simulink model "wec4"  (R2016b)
settings: Solver=ode4  StartTime=0  StopTime=1000  FixedStep=0.005  MaxStep=0.005  RelTol=1e-3  EnableMultiTasking=on
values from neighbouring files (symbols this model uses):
  arAdaptiveLawData = 1/2*zModelSimple.zModelPto.arFreq.*     zModelSimple.zModelPto.arMagnitude./     cos(zModelSimple.zModelPto.arPhase*pi/180+pi/2)    [IMPACT_Control.m]
  arAdaptiveLawDataX = 1/2*zModelSimpleX.zModelPto.arFreq.*         zModelSimpleX.zModelPto.arMagnitude./         cos(zModelSimpleX.zModelPto.arPhase*pi/180+pi/2)    [IMPACT_Control.m]
  arControllerRampGain = [0,0,1,1]    [IMPACT_Control.m]
  arControllerRampTime = [0 rStartRampTime rStartRampTime+rRampTimeLength 8000]    [IMPACT_Control.m]
  arEkfInitialisation = zeros(1,11)    [IMPACT_Control.m]
  arEkfInitialisationX = zeros(1,11)    [IMPACT_Control.m]
  arFrequency = zModelSimple.zModelPto.arFreq    [IMPACT_Control.m]
  arFrequencyRange = zModelSimple.zModelPto.arFreq    [IMPACT_Control.m]
  arFrequencyX = zModelSimpleX.zModelPto.arFreq    [IMPACT_Control.m]
  arImpedance = 1./zModelSimple.zModelPto.arMagnitude./zModelSimple.zModelPto.arFreq    [IMPACT_Control.m]
  arImpedanceX = 1./zModelSimpleX.zModelPto.arMagnitude./zModelSimpleX.zModelPto.arFreq    [IMPACT_Control.m]
  CentralPTOPreload = -1.6113e+07    (= -16113000)    [wecSimInputFile.m]
  F1 = [4.243 2.375 -12.243]    [wecSimInputFile.m]
  F2 = [4.243 -2.375 -12.243]    [wecSimInputFile.m]
  F3 = [-4.243 -2.375 -12.243]    [wecSimInputFile.m]
  F4 = [-4.243 2.375 -12.243]    [wecSimInputFile.m]
  FC = [0 0 -14]    [wecSimInputFile.m]
  iAdaptiveDamping = 0    [wec4IMPACT_Project.m]    (also in IMPACT_Control.m = handles.iAdaptiveDamping; wec1_IMPACT_Project.m; wec2_IMPACT_Project.m; wec3_IMPACT_Project.m)
  iControlType = 2    [wec4IMPACT_Project.m]    (also in IMPACT_Control.m = handles.iControlType; wec1_IMPACT_Project.m = 1; wec2_IMPACT_Project.m = 1; wec3_IMPACT_Project.m = 1)
  iPtoPositionConstraint = 1    [wec4IMPACT_Project.m]    (also in IMPACT_Control.m = handles.iPtoPositionConstraint; wec1_IMPACT_Project.m = 0; wec2_IMPACT_Project.m; wec3_IMPACT_Project.m)
  iSensorNoise = 0    [IMPACT_Control.m]
  m = m+1    (= 2)    [checkParamFile.m]
  PTOrotation = atan((T1(2)-F1(2))/(T1(1)-F1(1)))    [wecSimInputFile.m]
  rCogFloater = -8    [wec4_IMPACT_Model.m]    (also in paramInitial.m = get( handles.edit_rCogFloater, 'String' ); wec1_IMPACT_Model.m = -18; wec2_IMPACT_Model.m = -8.5; wec3_IMPACT_Model.m = -0.7)
  rCogSpar = -36.6    [wec4_IMPACT_Model.m]    (also in paramInitial.m = get( handles.edit_rCogSpar, 'String' ); wec3_IMPACT_Model.m = -21.3; wec3_IMPACT_Model2.m = -21.3)
  rDisplacementLimit = 10.000000    (= 10)    [wec4IMPACT_Project.m]    (also in IMPACT_Control.m = getValue(handles.edit_displacementLimit); wec1_IMPACT_Project.m; wec2_IMPACT_Project.m; wec3_IMPACT_Project.m = 3)
  rDisplacementLimitX = 10.000000    (= 10)    [wec4IMPACT_Project.m]    (also in IMPACT_Control.m = getValue(handles.edit_displacementLimitX); wec1_IMPACT_Project.m = 0; wec2_IMPACT_Project.m; wec3_IMPACT_Project.m = 0)
  rGainForAntiWIndUp = tfControllerDiscrete.rGain    [IMPACT_Control.m]
  rGainForAntiWIndUpX = tfControllerXDiscrete.rGain    [IMPACT_Control.m]
  rMaxForcePto = 300000000.000000    (= 300000000)    [wec4IMPACT_Project.m]    (also in IMPACT_Control.m = getValue(handles.edit_maxForcePto); wec1_IMPACT_Project.m = 1e+15; wec2_IMPACT_Project.m = 1e+15; wec3_IMPACT_Project.m = 1000000000)
  rMinForcePto = -300000000.000000    (= -300000000)    [wec4IMPACT_Project.m]    (also in IMPACT_Control.m = getValue(handles.edit_minForcePto); wec1_IMPACT_Project.m = -1e+15; wec2_IMPACT_Project.m = -1e+15; wec3_IMPACT_Project.m = -1000000000)
  rMooringX = 20000    [wec4_IMPACT_Model.m]    (also in paramInitial.m = get( handles.edit_rMooringX, 'String' ); wec3_IMPACT_Model.m = 10000; wec3_IMPACT_Model2.m = 10000)
  rMooringZ = 10000    [wec4_IMPACT_Model.m]    (also in paramInitial.m = get( handles.edit_rMooringZ, 'String' ); wec3_IMPACT_Model.m = 0; wec3_IMPACT_Model2.m = 0)
  rOutputSampleTime = 0.010000    (= 0.01)    [wec4IMPACT_Project.m]    (also in IMPACT_Control.m = getValue(handles.edit_outputSampleTime); wec1_IMPACT_Project.m; wec2_IMPACT_Project.m; wec3_IMPACT_Project.m)
  rPassiveDampingGain = -604830.000000    (= -604830)    [wec4IMPACT_Project.m]    (also in IMPACT_Control.m = getValue(handles.edit_gainPLD); wec1_IMPACT_Project.m = -214018.1537; wec2_IMPACT_Project.m = -1948070; wec3_IMPACT_Project.m = -519390)
  rPassiveDampingGainX = -278660.000000    (= -278660)    [wec4IMPACT_Project.m]    (also in IMPACT_Control.m = getValue(handles.edit_gainPLDX); wec1_IMPACT_Project.m = 0; wec2_IMPACT_Project.m = 0; wec3_IMPACT_Project.m = 0)
  rTetherPretension = 1.6113e+07    (= 16113000)    [wec4_IMPACT_Model.m]    (also in paramInitial.m = get( handles.edit_rTetherPretension, 'String' ); wec3_IMPACT_Model.m = 0; wec3_IMPACT_Model2.m = 0)
  rTetherSpring = 500000    [wec4_IMPACT_Model.m]    (also in paramInitial.m = get( handles.edit_rTetherSpring, 'String' ); wec3_IMPACT_Model.m = 0; wec3_IMPACT_Model2.m = 0)
  rUpperFrequencyLimit = EKFFloater.upperFreq    [IMPACT_Control.m]
  rXf = 4.243    [wec4AdditionalParams.m]
  rXs = 16.075    [wec4AdditionalParams.m]
  rYf = 2.375    [wec4AdditionalParams.m]
  rYs = 16.075    [wec4AdditionalParams.m]
  rZf = 4.243    [wec4AdditionalParams.m]
  rZs = 2.4350    (= 2.435)    [wec4AdditionalParams.m]
  rZTetherF = 6    [wec4AdditionalParams.m]
  rZTetherS = 2.4350    (= 2.435)    [wec4AdditionalParams.m]
  s = tf('s')    [wec4_IMPACT_Model.m]    (also in IMPACT_Control.m; wec1_IMPACT_Model.m; wec2_IMPACT_Model.m; wec3_IMPACT_Model.m)
  SidePTO1Preload = PreloadPTOCorner    (= 0)    [wecSimInputFile.m]
  SidePTO2Preload = PreloadPTOCorner    (= 0)    [wecSimInputFile.m]
  SidePTO3Preload = PreloadPTOCorner    (= 0)    [wecSimInputFile.m]
  SidePTO4Preload = PreloadPTOCorner    (= 0)    [wecSimInputFile.m]
  simu = simulationClass()    [wecSimInputFile.m]
  T1 = [16.075 16.075 -34.165]    [wecSimInputFile.m]
  T2 = [16.075 -16.075 -34.165]    [wecSimInputFile.m]
  T3 = [-16.075 -16.075 -34.165]    [wecSimInputFile.m]
  T4 = [-16.075 16.075 -34.165]    [wecSimInputFile.m]
  TC = [0 0 -34.165]    [wecSimInputFile.m]
  waves = waveClass('irregular')    [wecSimInputFile.m]
  Z = magPhaseToComplex(zModelTf)    [IMPACT_Control.m]
undefined symbols (not defined in the file or in its folder): arControllerDiscreteDen, arControllerDiscreteNum, arControllerDiscreteXDen, arControllerDiscreteXNum, arExcForceFloaterDen, arExcForceFloaterNum, arExcForceFloaterXDen, arExcForceFloaterXNum, arExcForceSparDen, arExcForceSparNum, arExcForceSparXDen, arExcForceSparXNum, arFexcFloaterDen, arFexcFloaterNum, arFexcFloaterXDen, arFexcFloaterXNum, arFexcSparDen, arFexcSparNum, arFexcSparXDen, arFexcSparXNum, Body, body, constraint, CTTime, deg, Elements, geometry, IRKB, kg, lenJ, mooring, N, pto, rAccelerationGainFloater, rAccelerationGainFloaterX, rAccelerationGainSpar, rAccelerationGainSparX, rad, rBuoyancyGainFloater, rBuoyancyGainFloaterX, rBuoyancyGainSpar, rBuoyancyGainSparX, rDampingGainFloater, rDampingGainFloaterX, rDampingGainSpar, rDampingGainSparX, Rigid, rMaxFocePto, wec4_float, wec4_reactor, WECSim_Lib, X, Y
libraries: nesl_utility x380, sm_lib x170, vrlib x91, simulink x12, WECSim_Lib x4
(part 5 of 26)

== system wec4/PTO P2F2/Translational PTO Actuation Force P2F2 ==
  Force : Inport
  Assignment{,1..3} (4 alike) : Assignment  IndexOptions=Index vector (dialog)  Indices=3  OutputSizes=1
  Bus Creator2 : BusCreator  Inputs=3
  Constant{,1..3} (4 alike) : Constant  Value=[0 0 0 0 0 0]
  InternalMechanics : Subsystem
  Mux : Mux  Inputs=2
  Mux1 : Mux  Inputs=2
  Mux2 : Mux  Inputs=8
  PS-Simulink Converter{,1..7} (8 alike) : nesl_utility/PS-Simulink Converter  PhysicalDomain=network_engine_domain  SubClassName=ps_output  LeftPortType=input  RightPortType=output  PseudoPeriodic=off  Frequencies=[]  Unit=1  AffineConversion=off
  Rigid Transform (Position) : sm_lib/Frames and Transforms/Rigid Transform  TranslationMethod=Cartesian  TranslationStandardOffset=0  TranslationLengthUnit=m  TranslationStandardAxis=+Z  TranslationCartesianOffset=pto.initDisp.initLinDisp + pto.loc  TranslationROffset=0  TranslationROffsetUnits=m  TranslationZOffset=0  TranslationZOffsetUnits=m  TranslationThetaOffset=0  TranslationThetaOffsetUnits=deg  RotationMethod=None  RotationAngleUnits=rad  RotationStandardAxis=+Y  RotationAngle=0  RotationArbitraryAxis=[0 1 0]  FollAlignAxisA=+X  BaseAlignAxisA=+Y  FollAlignAxisB=+Y  BaseAlignAxisB=+Z  RotationSequenceAxes=FollowerAxes  RotationSequence=XYX  RotationSequenceAngles=[0 0 0]  RotationSequenceAnglesUnits=deg  RotationMatrix=[1 0 0; 0 1 0; 0 0 1]
  Rigid Transform (Position)1 : sm_lib/Frames and Transforms/Rigid Transform  TranslationMethod=Cartesian  TranslationStandardOffset=0  TranslationLengthUnit=m  TranslationStandardAxis=+Z  TranslationCartesianOffset=pto.initDisp.initLinDisp + pto.loc  TranslationROffset=0  TranslationROffsetUnits=m  TranslationZOffset=0  TranslationZOffsetUnits=m  TranslationThetaOffset=0  TranslationThetaOffsetUnits=deg  RotationMethod=None  RotationAngleUnits=rad  RotationStandardAxis=+Y  RotationAngle=0  RotationArbitraryAxis=[0 1 0]  FollAlignAxisA=+X  BaseAlignAxisA=+Y  FollAlignAxisB=+Y  BaseAlignAxisB=+Z  RotationSequenceAxes=FollowerAxes  RotationSequence=XYX  RotationSequenceAngles=[0 0 0]  RotationSequenceAnglesUnits=deg  RotationMatrix=[1 0 0; 0 1 0; 0 0 1]
  Rigid Transform (Orientation) : sm_lib/Frames and Transforms/Rigid Transform  TranslationMethod=None  TranslationStandardOffset=0  TranslationLengthUnit=m  TranslationStandardAxis=+Z  TranslationCartesianOffset=0  TranslationROffset=0  TranslationROffsetUnits=m  TranslationZOffset=0  TranslationZOffsetUnits=m  TranslationThetaOffset=0  TranslationThetaOffsetUnits=deg  RotationMethod=RotationMatrix  RotationAngleUnits=rad  RotationStandardAxis=+Y  RotationAngle=0  RotationArbitraryAxis=[0 1 0]  FollAlignAxisA=+X  BaseAlignAxisA=+Y  FollAlignAxisB=+Y  BaseAlignAxisB=+Z  RotationSequenceAxes=FollowerAxes  RotationSequence=XYX  RotationSequenceAngles=[0 0 0]  RotationSequenceAnglesUnits=deg  RotationMatrix=pto.orientation.rotationMatrix
  Rigid Transform (Orientation)1 : sm_lib/Frames and Transforms/Rigid Transform  TranslationMethod=None  TranslationStandardOffset=0  TranslationLengthUnit=m  TranslationStandardAxis=+Z  TranslationCartesianOffset=0  TranslationROffset=0  TranslationROffsetUnits=m  TranslationZOffset=0  TranslationZOffsetUnits=m  TranslationThetaOffset=0  TranslationThetaOffsetUnits=deg  RotationMethod=RotationMatrix  RotationAngleUnits=rad  RotationStandardAxis=+Y  RotationAngle=0  RotationArbitraryAxis=[0 1 0]  FollAlignAxisA=+X  BaseAlignAxisA=+Y  FollAlignAxisB=+Y  BaseAlignAxisB=+Z  RotationSequenceAxes=FollowerAxes  RotationSequence=XYX  RotationSequenceAngles=[0 0 0]  RotationSequenceAnglesUnits=deg  RotationMatrix=pto.orientation.rotationMatrix
  Simulink-PS Converter : nesl_utility/Simulink-PS Converter  PhysicalDomain=network_engine_domain  SubClassName=ps_input  LeftPortType=input  RightPortType=output  PseudoPeriodic=off  Frequencies=[]  NoiseDistribution=none  NoiseParameters=[]  Unit=1  AffineConversion=off  InputFiltering=off  SimscapeFilterOrder=1  InputFilterTimeConstant=0.001  UdotUserProvided=1
  Translational PCC (Prismatic Joint) : sm_lib/Joints/Prismatic Joint  SenseConstraintForce=on  SenseConstraintForceX=off  SenseConstraintForceY=off  SenseConstraintForceZ=off  SenseConstraintTorque=on  SenseConstraintTorqueX=off  SenseConstraintTorqueY=off  SenseConstraintTorqueZ=off  SenseTotalForce=on  SenseTotalForceX=off  SenseTotalForceY=off  SenseTotalForceZ=off  SenseTotalTorque=on  SenseTotalTorqueX=off  SenseTotalTorqueY=off  SenseTotalTorqueZ=off  CompositeWrenchDir=BaseOnFollower  CompositeWrenchFrame=BaseFrame  EquilibriumPosition=0  EquilibriumPositionUnits=m  SpringStiffness=pto.k  SpringStiffnessUnits=N/m  DampingCoefficient=pto.c  DampingCoefficientUnits=N/(m/s)  TorqueActuationMode=InputTorque  MotionActuationMode=ComputedMotion  SensePosition=on  SenseVelocity=on  SenseAcceleration=on  SenseTorqueForce=on  PositionTargetSpecify=off  PositionTargetPriority=High  PositionTargetValue=0  PositionTargetValueUnits=m  VelocityTargetSpecify=off  VelocityTargetPriority=High  VelocityTargetValue=0  VelocityTargetValueUnits=m/s
  output : ToWorkspace  VariableName=pto2_out  SaveFormat=Structure With Time  SampleTime=-1
  F : PMIOPort  Port=1  Side=Right
  B : PMIOPort  Port=2  Side=Left
  Response : Outport
  ptoForce : Outport  Port=2
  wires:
  Bus Creator2/1 -> Response/1
  Assignment/1 -> Mux2/1, Bus Creator2/1, InternalMechanics/1(Position)  "position"
  Assignment1/1 -> Mux2/2, Bus Creator2/2, InternalMechanics/2(Velocity)  "velocity"
  Assignment2/1 -> Mux2/3, Bus Creator2/3  "acceleration"
  Force/1 -> Simulink-PS Converter/1
  Mux2/1 -> output/1
  Mux/1 -> Mux2/6  "forceConstraint"
  Mux1/1 -> Mux2/4  "forceTotal"
  PS-Simulink Converter4/1 -> Mux/1
  PS-Simulink Converter5/1 -> Mux/2
  PS-Simulink Converter6/1 -> Mux1/1
  PS-Simulink Converter7/1 -> Mux1/2
  Constant/1 -> Assignment/1
  PS-Simulink Converter/1 -> Assignment/2
  Constant1/1 -> Assignment1/1
  PS-Simulink Converter1/1 -> Assignment1/2
  Constant2/1 -> Assignment2/1
  PS-Simulink Converter2/1 -> Assignment2/2
  InternalMechanics/1(Force) -> Mux2/7  "forceInternalMechanics"
  InternalMechanics/2(Power) -> Mux2/8  "powerInternalMechanics"
  Constant3/1 -> Assignment3/1
  PS-Simulink Converter3/1 -> Assignment3/2  "forceActuation"
  Assignment3/1 -> ptoForce/1, Mux2/5  "forceActuation"
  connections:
  Rigid Transform (Position)/RConn1 -- Rigid Transform (Orientation)/LConn1
  Rigid Transform (Position)1/RConn1 -- Rigid Transform (Orientation)1/LConn1
  Simulink-PS Converter/RConn1 -- Translational PCC (Prismatic Joint)/LConn2
  Rigid Transform (Orientation)/RConn1 -- Translational PCC (Prismatic Joint)/LConn1
  Rigid Transform (Position)/LConn1 -- B/RConn1
  Translational PCC (Prismatic Joint)/RConn5 -- PS-Simulink Converter3/LConn1
  Translational PCC (Prismatic Joint)/RConn9 -- PS-Simulink Converter7/LConn1
  Rigid Transform (Orientation)1/RConn1 -- Translational PCC (Prismatic Joint)/RConn1
  Translational PCC (Prismatic Joint)/RConn4 -- PS-Simulink Converter2/LConn1
  Translational PCC (Prismatic Joint)/RConn7 -- PS-Simulink Converter5/LConn1
  Translational PCC (Prismatic Joint)/RConn3 -- PS-Simulink Converter1/LConn1
  Rigid Transform (Position)1/LConn1 -- F/RConn1
  Translational PCC (Prismatic Joint)/RConn8 -- PS-Simulink Converter6/LConn1
  Translational PCC (Prismatic Joint)/RConn2 -- PS-Simulink Converter/LConn1
  Translational PCC (Prismatic Joint)/RConn6 -- PS-Simulink Converter4/LConn1

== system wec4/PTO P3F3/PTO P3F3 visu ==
  note: 1) Add Subsystem or Model blocks as valid variant choices. 2) You cannot connect blocks at this level. At simulation, connectivity is automatically determined, based on the active variant and port name matching.
  Hydrodynamic Body : Subsystem  VariantControl=sv_b6_hydroBody
  Non-Hydro Body : Subsystem  VariantControl=sv_b6_nonHydroBody
  Conn : PMIOPort  Port=1  Side=Right

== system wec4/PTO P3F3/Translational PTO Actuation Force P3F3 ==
  Force : Inport
  Assignment{,1..3} (4 alike) : Assignment  IndexOptions=Index vector (dialog)  Indices=3  OutputSizes=1
  Bus Creator2 : BusCreator  Inputs=3
  Constant{,1..3} (4 alike) : Constant  Value=[0 0 0 0 0 0]
  InternalMechanics : Subsystem
  Mux : Mux  Inputs=2
  Mux1 : Mux  Inputs=2
  Mux2 : Mux  Inputs=8
  PS-Simulink Converter{,1..7} (8 alike) : nesl_utility/PS-Simulink Converter  PhysicalDomain=network_engine_domain  SubClassName=ps_output  LeftPortType=input  RightPortType=output  PseudoPeriodic=off  Frequencies=[]  Unit=1  AffineConversion=off
  Rigid Transform (Position) : sm_lib/Frames and Transforms/Rigid Transform  TranslationMethod=Cartesian  TranslationStandardOffset=0  TranslationLengthUnit=m  TranslationStandardAxis=+Z  TranslationCartesianOffset=pto.initDisp.initLinDisp + pto.loc  TranslationROffset=0  TranslationROffsetUnits=m  TranslationZOffset=0  TranslationZOffsetUnits=m  TranslationThetaOffset=0  TranslationThetaOffsetUnits=deg  RotationMethod=None  RotationAngleUnits=rad  RotationStandardAxis=+Y  RotationAngle=0  RotationArbitraryAxis=[0 1 0]  FollAlignAxisA=+X  BaseAlignAxisA=+Y  FollAlignAxisB=+Y  BaseAlignAxisB=+Z  RotationSequenceAxes=FollowerAxes  RotationSequence=XYX  RotationSequenceAngles=[0 0 0]  RotationSequenceAnglesUnits=deg  RotationMatrix=[1 0 0; 0 1 0; 0 0 1]
  Rigid Transform (Position)1 : sm_lib/Frames and Transforms/Rigid Transform  TranslationMethod=Cartesian  TranslationStandardOffset=0  TranslationLengthUnit=m  TranslationStandardAxis=+Z  TranslationCartesianOffset=pto.initDisp.initLinDisp + pto.loc  TranslationROffset=0  TranslationROffsetUnits=m  TranslationZOffset=0  TranslationZOffsetUnits=m  TranslationThetaOffset=0  TranslationThetaOffsetUnits=deg  RotationMethod=None  RotationAngleUnits=rad  RotationStandardAxis=+Y  RotationAngle=0  RotationArbitraryAxis=[0 1 0]  FollAlignAxisA=+X  BaseAlignAxisA=+Y  FollAlignAxisB=+Y  BaseAlignAxisB=+Z  RotationSequenceAxes=FollowerAxes  RotationSequence=XYX  RotationSequenceAngles=[0 0 0]  RotationSequenceAnglesUnits=deg  RotationMatrix=[1 0 0; 0 1 0; 0 0 1]
  Rigid Transform (Orientation) : sm_lib/Frames and Transforms/Rigid Transform  TranslationMethod=None  TranslationStandardOffset=0  TranslationLengthUnit=m  TranslationStandardAxis=+Z  TranslationCartesianOffset=0  TranslationROffset=0  TranslationROffsetUnits=m  TranslationZOffset=0  TranslationZOffsetUnits=m  TranslationThetaOffset=0  TranslationThetaOffsetUnits=deg  RotationMethod=RotationMatrix  RotationAngleUnits=rad  RotationStandardAxis=+Y  RotationAngle=0  RotationArbitraryAxis=[0 1 0]  FollAlignAxisA=+X  BaseAlignAxisA=+Y  FollAlignAxisB=+Y  BaseAlignAxisB=+Z  RotationSequenceAxes=FollowerAxes  RotationSequence=XYX  RotationSequenceAngles=[0 0 0]  RotationSequenceAnglesUnits=deg  RotationMatrix=pto.orientation.rotationMatrix
  Rigid Transform (Orientation)1 : sm_lib/Frames and Transforms/Rigid Transform  TranslationMethod=None  TranslationStandardOffset=0  TranslationLengthUnit=m  TranslationStandardAxis=+Z  TranslationCartesianOffset=0  TranslationROffset=0  TranslationROffsetUnits=m  TranslationZOffset=0  TranslationZOffsetUnits=m  TranslationThetaOffset=0  TranslationThetaOffsetUnits=deg  RotationMethod=RotationMatrix  RotationAngleUnits=rad  RotationStandardAxis=+Y  RotationAngle=0  RotationArbitraryAxis=[0 1 0]  FollAlignAxisA=+X  BaseAlignAxisA=+Y  FollAlignAxisB=+Y  BaseAlignAxisB=+Z  RotationSequenceAxes=FollowerAxes  RotationSequence=XYX  RotationSequenceAngles=[0 0 0]  RotationSequenceAnglesUnits=deg  RotationMatrix=pto.orientation.rotationMatrix
  Simulink-PS Converter : nesl_utility/Simulink-PS Converter  PhysicalDomain=network_engine_domain  SubClassName=ps_input  LeftPortType=input  RightPortType=output  PseudoPeriodic=off  Frequencies=[]  NoiseDistribution=none  NoiseParameters=[]  Unit=1  AffineConversion=off  InputFiltering=off  SimscapeFilterOrder=1  InputFilterTimeConstant=0.001  UdotUserProvided=1
  Translational PCC (Prismatic Joint) : sm_lib/Joints/Prismatic Joint  SenseConstraintForce=on  SenseConstraintForceX=off  SenseConstraintForceY=off  SenseConstraintForceZ=off  SenseConstraintTorque=on  SenseConstraintTorqueX=off  SenseConstraintTorqueY=off  SenseConstraintTorqueZ=off  SenseTotalForce=on  SenseTotalForceX=off  SenseTotalForceY=off  SenseTotalForceZ=off  SenseTotalTorque=on  SenseTotalTorqueX=off  SenseTotalTorqueY=off  SenseTotalTorqueZ=off  CompositeWrenchDir=BaseOnFollower  CompositeWrenchFrame=BaseFrame  EquilibriumPosition=0  EquilibriumPositionUnits=m  SpringStiffness=pto.k  SpringStiffnessUnits=N/m  DampingCoefficient=pto.c  DampingCoefficientUnits=N/(m/s)  TorqueActuationMode=InputTorque  MotionActuationMode=ComputedMotion  SensePosition=on  SenseVelocity=on  SenseAcceleration=on  SenseTorqueForce=on  PositionTargetSpecify=off  PositionTargetPriority=High  PositionTargetValue=0  PositionTargetValueUnits=m  VelocityTargetSpecify=off  VelocityTargetPriority=High  VelocityTargetValue=0  VelocityTargetValueUnits=m/s
  output : ToWorkspace  VariableName=pto3_out  SaveFormat=Structure With Time  SampleTime=-1
  F : PMIOPort  Port=1  Side=Right
  B : PMIOPort  Port=2  Side=Left
  Response : Outport
  ptoForce : Outport  Port=2
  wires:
  Bus Creator2/1 -> Response/1
  Assignment/1 -> Mux2/1, Bus Creator2/1, InternalMechanics/1(Position)  "position"
  Assignment1/1 -> Mux2/2, Bus Creator2/2, InternalMechanics/2(Velocity)  "velocity"
  Assignment2/1 -> Mux2/3, Bus Creator2/3  "acceleration"
  Force/1 -> Simulink-PS Converter/1
  Mux2/1 -> output/1
  Mux/1 -> Mux2/6  "forceConstraint"
  Mux1/1 -> Mux2/4  "forceTotal"
  PS-Simulink Converter4/1 -> Mux/1
  PS-Simulink Converter5/1 -> Mux/2
  PS-Simulink Converter6/1 -> Mux1/1
  PS-Simulink Converter7/1 -> Mux1/2
  Constant/1 -> Assignment/1
  PS-Simulink Converter/1 -> Assignment/2
  Constant1/1 -> Assignment1/1
  PS-Simulink Converter1/1 -> Assignment1/2
  Constant2/1 -> Assignment2/1
  PS-Simulink Converter2/1 -> Assignment2/2
  InternalMechanics/1(Force) -> Mux2/7  "forceInternalMechanics"
  InternalMechanics/2(Power) -> Mux2/8  "powerInternalMechanics"
  Constant3/1 -> Assignment3/1
  PS-Simulink Converter3/1 -> Assignment3/2  "forceActuation"
  Assignment3/1 -> ptoForce/1, Mux2/5  "forceActuation"
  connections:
  Rigid Transform (Position)/RConn1 -- Rigid Transform (Orientation)/LConn1
  Rigid Transform (Position)1/RConn1 -- Rigid Transform (Orientation)1/LConn1
  Simulink-PS Converter/RConn1 -- Translational PCC (Prismatic Joint)/LConn2
  Rigid Transform (Orientation)/RConn1 -- Translational PCC (Prismatic Joint)/LConn1
  Rigid Transform (Position)/LConn1 -- B/RConn1
  Translational PCC (Prismatic Joint)/RConn5 -- PS-Simulink Converter3/LConn1
  Translational PCC (Prismatic Joint)/RConn9 -- PS-Simulink Converter7/LConn1
  Rigid Transform (Orientation)1/RConn1 -- Translational PCC (Prismatic Joint)/RConn1
  Translational PCC (Prismatic Joint)/RConn4 -- PS-Simulink Converter2/LConn1
  Translational PCC (Prismatic Joint)/RConn7 -- PS-Simulink Converter5/LConn1
  Translational PCC (Prismatic Joint)/RConn3 -- PS-Simulink Converter1/LConn1
  Rigid Transform (Position)1/LConn1 -- F/RConn1
  Translational PCC (Prismatic Joint)/RConn8 -- PS-Simulink Converter6/LConn1
  Translational PCC (Prismatic Joint)/RConn2 -- PS-Simulink Converter/LConn1
  Translational PCC (Prismatic Joint)/RConn6 -- PS-Simulink Converter4/LConn1

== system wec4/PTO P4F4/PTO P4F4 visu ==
  note: 1) Add Subsystem or Model blocks as valid variant choices. 2) You cannot connect blocks at this level. At simulation, connectivity is automatically determined, based on the active variant and port name matching.
  Hydrodynamic Body : Subsystem  VariantControl=sv_b7_hydroBody
  Non-Hydro Body : Subsystem  VariantControl=sv_b7_nonHydroBody
  Conn : PMIOPort  Port=1  Side=Right

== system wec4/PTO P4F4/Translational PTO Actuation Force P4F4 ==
  Force : Inport
  Assignment{,1..3} (4 alike) : Assignment  IndexOptions=Index vector (dialog)  Indices=3  OutputSizes=1
  Bus Creator2 : BusCreator  Inputs=3
  Constant{,1..3} (4 alike) : Constant  Value=[0 0 0 0 0 0]
  InternalMechanics : Subsystem
  Mux : Mux  Inputs=2
  Mux1 : Mux  Inputs=2
  Mux2 : Mux  Inputs=8
  PS-Simulink Converter{,1..7} (8 alike) : nesl_utility/PS-Simulink Converter  PhysicalDomain=network_engine_domain  SubClassName=ps_output  LeftPortType=input  RightPortType=output  PseudoPeriodic=off  Frequencies=[]  Unit=1  AffineConversion=off
  Rigid Transform (Position) : sm_lib/Frames and Transforms/Rigid Transform  TranslationMethod=Cartesian  TranslationStandardOffset=0  TranslationLengthUnit=m  TranslationStandardAxis=+Z  TranslationCartesianOffset=pto.initDisp.initLinDisp + pto.loc  TranslationROffset=0  TranslationROffsetUnits=m  TranslationZOffset=0  TranslationZOffsetUnits=m  TranslationThetaOffset=0  TranslationThetaOffsetUnits=deg  RotationMethod=None  RotationAngleUnits=rad  RotationStandardAxis=+Y  RotationAngle=0  RotationArbitraryAxis=[0 1 0]  FollAlignAxisA=+X  BaseAlignAxisA=+Y  FollAlignAxisB=+Y  BaseAlignAxisB=+Z  RotationSequenceAxes=FollowerAxes  RotationSequence=XYX  RotationSequenceAngles=[0 0 0]  RotationSequenceAnglesUnits=deg  RotationMatrix=[1 0 0; 0 1 0; 0 0 1]
  Rigid Transform (Position)1 : sm_lib/Frames and Transforms/Rigid Transform  TranslationMethod=Cartesian  TranslationStandardOffset=0  TranslationLengthUnit=m  TranslationStandardAxis=+Z  TranslationCartesianOffset=pto.initDisp.initLinDisp + pto.loc  TranslationROffset=0  TranslationROffsetUnits=m  TranslationZOffset=0  TranslationZOffsetUnits=m  TranslationThetaOffset=0  TranslationThetaOffsetUnits=deg  RotationMethod=None  RotationAngleUnits=rad  RotationStandardAxis=+Y  RotationAngle=0  RotationArbitraryAxis=[0 1 0]  FollAlignAxisA=+X  BaseAlignAxisA=+Y  FollAlignAxisB=+Y  BaseAlignAxisB=+Z  RotationSequenceAxes=FollowerAxes  RotationSequence=XYX  RotationSequenceAngles=[0 0 0]  RotationSequenceAnglesUnits=deg  RotationMatrix=[1 0 0; 0 1 0; 0 0 1]
  Rigid Transform (Orientation) : sm_lib/Frames and Transforms/Rigid Transform  TranslationMethod=None  TranslationStandardOffset=0  TranslationLengthUnit=m  TranslationStandardAxis=+Z  TranslationCartesianOffset=0  TranslationROffset=0  TranslationROffsetUnits=m  TranslationZOffset=0  TranslationZOffsetUnits=m  TranslationThetaOffset=0  TranslationThetaOffsetUnits=deg  RotationMethod=RotationMatrix  RotationAngleUnits=rad  RotationStandardAxis=+Y  RotationAngle=0  RotationArbitraryAxis=[0 1 0]  FollAlignAxisA=+X  BaseAlignAxisA=+Y  FollAlignAxisB=+Y  BaseAlignAxisB=+Z  RotationSequenceAxes=FollowerAxes  RotationSequence=XYX  RotationSequenceAngles=[0 0 0]  RotationSequenceAnglesUnits=deg  RotationMatrix=pto.orientation.rotationMatrix
  Rigid Transform (Orientation)1 : sm_lib/Frames and Transforms/Rigid Transform  TranslationMethod=None  TranslationStandardOffset=0  TranslationLengthUnit=m  TranslationStandardAxis=+Z  TranslationCartesianOffset=0  TranslationROffset=0  TranslationROffsetUnits=m  TranslationZOffset=0  TranslationZOffsetUnits=m  TranslationThetaOffset=0  TranslationThetaOffsetUnits=deg  RotationMethod=RotationMatrix  RotationAngleUnits=rad  RotationStandardAxis=+Y  RotationAngle=0  RotationArbitraryAxis=[0 1 0]  FollAlignAxisA=+X  BaseAlignAxisA=+Y  FollAlignAxisB=+Y  BaseAlignAxisB=+Z  RotationSequenceAxes=FollowerAxes  RotationSequence=XYX  RotationSequenceAngles=[0 0 0]  RotationSequenceAnglesUnits=deg  RotationMatrix=pto.orientation.rotationMatrix
  Simulink-PS Converter : nesl_utility/Simulink-PS Converter  PhysicalDomain=network_engine_domain  SubClassName=ps_input  LeftPortType=input  RightPortType=output  PseudoPeriodic=off  Frequencies=[]  NoiseDistribution=none  NoiseParameters=[]  Unit=1  AffineConversion=off  InputFiltering=off  SimscapeFilterOrder=1  InputFilterTimeConstant=0.001  UdotUserProvided=1
  Translational PCC (Prismatic Joint) : sm_lib/Joints/Prismatic Joint  SenseConstraintForce=on  SenseConstraintForceX=off  SenseConstraintForceY=off  SenseConstraintForceZ=off  SenseConstraintTorque=on  SenseConstraintTorqueX=off  SenseConstraintTorqueY=off  SenseConstraintTorqueZ=off  SenseTotalForce=on  SenseTotalForceX=off  SenseTotalForceY=off  SenseTotalForceZ=off  SenseTotalTorque=on  SenseTotalTorqueX=off  SenseTotalTorqueY=off  SenseTotalTorqueZ=off  CompositeWrenchDir=BaseOnFollower  CompositeWrenchFrame=BaseFrame  EquilibriumPosition=0  EquilibriumPositionUnits=m  SpringStiffness=pto.k  SpringStiffnessUnits=N/m  DampingCoefficient=pto.c  DampingCoefficientUnits=N/(m/s)  TorqueActuationMode=InputTorque  MotionActuationMode=ComputedMotion  SensePosition=on  SenseVelocity=on  SenseAcceleration=on  SenseTorqueForce=on  PositionTargetSpecify=off  PositionTargetPriority=High  PositionTargetValue=0  PositionTargetValueUnits=m  VelocityTargetSpecify=off  VelocityTargetPriority=High  VelocityTargetValue=0  VelocityTargetValueUnits=m/s
  output : ToWorkspace  VariableName=pto4_out  SaveFormat=Structure With Time  SampleTime=-1
  F : PMIOPort  Port=1  Side=Right
  B : PMIOPort  Port=2  Side=Left
  Response : Outport
  ptoForce : Outport  Port=2
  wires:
  Bus Creator2/1 -> Response/1
  Assignment/1 -> Mux2/1, Bus Creator2/1, InternalMechanics/1(Position)  "position"
  Assignment1/1 -> Mux2/2, Bus Creator2/2, InternalMechanics/2(Velocity)  "velocity"
  Assignment2/1 -> Mux2/3, Bus Creator2/3  "acceleration"
  Force/1 -> Simulink-PS Converter/1
  Mux2/1 -> output/1
  Mux/1 -> Mux2/6  "forceConstraint"
  Mux1/1 -> Mux2/4  "forceTotal"
  PS-Simulink Converter4/1 -> Mux/1
  PS-Simulink Converter5/1 -> Mux/2
  PS-Simulink Converter6/1 -> Mux1/1
  PS-Simulink Converter7/1 -> Mux1/2
  Constant/1 -> Assignment/1
  PS-Simulink Converter/1 -> Assignment/2
  Constant1/1 -> Assignment1/1
  PS-Simulink Converter1/1 -> Assignment1/2
  Constant2/1 -> Assignment2/1
  PS-Simulink Converter2/1 -> Assignment2/2
  InternalMechanics/1(Force) -> Mux2/7  "forceInternalMechanics"
  InternalMechanics/2(Power) -> Mux2/8  "powerInternalMechanics"
  Constant3/1 -> Assignment3/1
  PS-Simulink Converter3/1 -> Assignment3/2  "forceActuation"
  Assignment3/1 -> ptoForce/1, Mux2/5  "forceActuation"
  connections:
  Rigid Transform (Position)/RConn1 -- Rigid Transform (Orientation)/LConn1
  Rigid Transform (Position)1/RConn1 -- Rigid Transform (Orientation)1/LConn1
  Simulink-PS Converter/RConn1 -- Translational PCC (Prismatic Joint)/LConn2
  Rigid Transform (Orientation)/RConn1 -- Translational PCC (Prismatic Joint)/LConn1
  Rigid Transform (Position)/LConn1 -- B/RConn1
  Translational PCC (Prismatic Joint)/RConn5 -- PS-Simulink Converter3/LConn1
  Translational PCC (Prismatic Joint)/RConn9 -- PS-Simulink Converter7/LConn1
  Rigid Transform (Orientation)1/RConn1 -- Translational PCC (Prismatic Joint)/RConn1
  Translational PCC (Prismatic Joint)/RConn4 -- PS-Simulink Converter2/LConn1
  Translational PCC (Prismatic Joint)/RConn7 -- PS-Simulink Converter5/LConn1
  Translational PCC (Prismatic Joint)/RConn3 -- PS-Simulink Converter1/LConn1
  Rigid Transform (Position)1/LConn1 -- F/RConn1
  Translational PCC (Prismatic Joint)/RConn8 -- PS-Simulink Converter6/LConn1
  Translational PCC (Prismatic Joint)/RConn2 -- PS-Simulink Converter/LConn1
  Translational PCC (Prismatic Joint)/RConn6 -- PS-Simulink Converter4/LConn1

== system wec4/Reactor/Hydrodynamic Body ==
  Additional Linear Damping Force Calculation : Subsystem
  B2B Subsystem : Subsystem  Variant=on
  Bus Creator : BusCreator  Inputs=6
  Bus Creator1 : BusCreator  Inputs=3
  Bus Selector1 : BusSelector  OutputSignals=F_Excitation,F_RadiationDamping,F_AddedMass,F_Restoring,F_MorrisonAndViscous,F_LinearDamping
  Bus Selector2 : BusSelector  OutputSignals=disp,vel,acc
  Hydrostatic Restoring Force Calculation : Subsystem
  Morrison Element and ViscousDampingForceCalculation : Subsystem
  Nonlinear Wave Elevation : Subsystem  TreatAsAtomicUnit=on  SystemSampleTime=simu.dtNL
  Structure : Subsystem
  Sum : Sum  Inputs=+-----
  To Workspace : ToWorkspace  VariableName=body2_out  SaveFormat=Structure With Time  SampleTime=-1
  Wave Diffraction and Excitation Force Calculation : Subsystem
  Wave Radiation Forces Calculation : Subsystem
  Conn : PMIOPort  Port=1  Side=Right
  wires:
  Additional Linear Damping Force Calculation/1(F_LinearDamping) -> Bus Creator/6
  Bus Creator/1 -> Bus Selector1/1, Bus Creator1/3  "BUS(7): Forces"
  Bus Selector2/1 -> [disp2]  "<disp>"
  Bus Selector2/3 -> [acc2]  "<acc>"
  Bus Selector2/2 -> [vel2]  "<vel>"
  Structure/1(Response) -> Bus Creator1/1, Bus Selector2/1
  Sum/1 -> Bus Creator1/2, Structure/1(Total Force)  "F_Total"
  Bus Creator1/1 -> To Workspace/1
  Bus Selector1/4 -> Sum/4  "<F_Restoring>"
  Bus Selector1/3 -> Sum/3  "<F_AddedMass>"
  Bus Selector1/5 -> Sum/5  "<F_MorrisonAndViscous>"
  Bus Selector1/2 -> Sum/2  "<F_RadiationDamping>"
  Bus Selector1/1 -> [Fex2], Sum/1  "<F_Excitation>"
  Bus Selector1/6 -> Sum/6  "<F_LinearDamping>"
  [acc2] -> B2B Subsystem/2(acc_in), Morrison Element and ViscousDampingForceCalculation/2(Acceleration)
  [vel2] -> Morrison Element and ViscousDampingForceCalculation/3(Velocity), Additional Linear Damping Force Calculation/1(Velocity), B2B Subsystem/1(vel_in)
  B2B Subsystem/2(acc) -> Wave Radiation Forces Calculation/2(Acceleration)
  B2B Subsystem/1(vel) -> Wave Radiation Forces Calculation/1(Velocity)
  [disp2] -> Hydrostatic Restoring Force Calculation/1(Displacement), Morrison Element and ViscousDampingForceCalculation/1(Displacement), Nonlinear Wave Elevation/1(Displacement), Wave Diffraction and Excitation Force Calculation/2(Displacement)
  Nonlinear Wave Elevation/1(Wave Elevation) -> Wave Diffraction and Excitation Force Calculation/3(WaveElv), Hydrostatic Restoring Force Calculation/2(Wave Elv)
  Hydrostatic Restoring Force Calculation/1(F_Restoring) -> Bus Creator/4
  Wave Radiation Forces Calculation/1(F_RadiationDamping) -> Bus Creator/2
  Wave Diffraction and Excitation Force Calculation/1(F_Excitation) -> Bus Creator/1
  Wave Radiation Forces Calculation/2(F_AddedMass) -> Bus Creator/3
  [Clock] -> Nonlinear Wave Elevation/2(Time), Wave Diffraction and Excitation Force Calculation/1(Time), Morrison Element and ViscousDampingForceCalculation/4(Time), Wave Radiation Forces Calculation/3(Time)
  Morrison Element and ViscousDampingForceCalculation/1(F_MorrisonAndViscous) -> Bus Creator/5
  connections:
  Conn/RConn1 -- Structure/RConn1

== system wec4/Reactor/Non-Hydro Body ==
  Bus Creator : BusCreator  Inputs=6
  Bus Creator1 : BusCreator  Inputs=3
  Bus Selector1 : BusSelector  OutputSignals=F_Excitation,F_RadiationDamping,F_AddedMass,F_Restoring,F_MorrisonAndViscous,F_LinearDamping
  Constant{,1..3,5} (5 alike) : Constant  Value=[0 0 0 0 0 0]
  Structure : Subsystem
  Sum : Sum  Inputs=+-----
  To Workspace : ToWorkspace  VariableName=body2_out  SaveFormat=Structure With Time  SampleTime=-1
  Weight and Buoyancy : Subsystem
  Conn : PMIOPort  Port=1  Side=Right
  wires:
  Bus Creator/1 -> Bus Creator1/3, Bus Selector1/1  "BUS(7): Forces"
  Structure/1(Response) -> Bus Creator1/1
  Sum/1 -> Bus Creator1/2, Structure/1(Total Force)  "F_Total"
  Bus Creator1/1 -> To Workspace/1
  Bus Selector1/4 -> Sum/4  "<F_Restoring>"
  Bus Selector1/3 -> Sum/3  "<F_AddedMass>"
  Bus Selector1/5 -> Sum/5  "<F_MorrisonAndViscous>"
  Bus Selector1/2 -> Sum/2  "<F_RadiationDamping>"
  Bus Selector1/1 -> Sum/1  "<F_Excitation>"
  Bus Selector1/6 -> Sum/6  "<F_LinearDamping>"
  Constant5/1 -> Bus Creator/6  "F_LinearDamping"
  Constant3/1 -> Bus Creator/5  "F_MorrisonAndViscous"
  Constant2/1 -> Bus Creator/3  "F_AddedMass"
  Constant1/1 -> Bus Creator/2  "F_RadiationDamping"
  Constant/1 -> Bus Creator/1  "F_Excitation"
  Weight and Buoyancy/1(Out1) -> Bus Creator/4  "F_Restoring"
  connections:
  Conn/RConn1 -- Structure/RConn1

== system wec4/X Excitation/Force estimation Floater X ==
  Acceleration : Inport
  Velocity : Inport  Port=2
  Position : Inport  Port=3
  PTO Force : Inport  Port=4
  Add : Sum  Inputs=+++
  Add1 : Sum  Inputs=++|
  Add2 : Sum  Inputs=++|
  Add3 : Sum  Inputs=++|
  Add4 : Sum  Inputs=|+-
  Band-Limited White Noise : simulink/Sources/Band-Limited White Noise  Cov=[0.1]  Ts=simu.dt  seed=[23341]
  Band-Limited White Noise1 : simulink/Sources/Band-Limited White Noise  Cov=[0.1]  Ts=simu.dt  seed=[23341]
  Band-Limited White Noise2 : simulink/Sources/Band-Limited White Noise  Cov=[0.1]  Ts=simu.dt  seed=[23341]
  Delay : Delay  DelayLength=1  SampleTime=simu.dt
  Gain : Gain  Gain=rAccelerationGainFloaterX
  Gain1 : Gain  Gain=rDampingGainFloaterX
  Gain2 : Gain  Gain=rBuoyancyGainFloaterX
  Gain3 : Gain  Gain=iSensorNoise
  Gain4 : Gain  Gain=iSensorNoise
  Gain5 : Gain  Gain=iSensorNoise
  To Workspace1 : ToWorkspace  VariableName=arInertialForceFloaterX  SampleTime=rOutputSampleTime
  To Workspace2 : ToWorkspace  VariableName=accComponentFlX  SampleTime=rOutputSampleTime
  To Workspace3 : ToWorkspace  VariableName=velComponentFlX  SampleTime=rOutputSampleTime
  To Workspace4 : ToWorkspace  VariableName=posComponentFlX  SampleTime=rOutputSampleTime
  To Workspace5 : ToWorkspace  VariableName=arPtoForceX  SampleTime=rOutputSampleTime
  Transfer Fcn : TransferFcn  Numerator=arExcForceFloaterXNum  Denominator=arExcForceFloaterXDen
  excForce : Outport
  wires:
  Transfer Fcn/1 -> Add4/1, To Workspace1/1
  Add4/1 -> excForce/1
  Add/1 -> Transfer Fcn/1
  Delay/1 -> Add4/2, To Workspace5/1
  Band-Limited White Noise2/1 -> Gain5/1
  Band-Limited White Noise1/1 -> Gain4/1
  Add1/1 -> Gain/1
  Velocity/1 -> Add3/2
  Gain3/1 -> Add1/1
  Add3/1 -> Gain1/1
  Gain4/1 -> Add3/1
  Gain/1 -> To Workspace2/1, Add/1
  Gain1/1 -> To Workspace3/1, Add/2
  Gain2/1 -> To Workspace4/1, Add/3
  PTO Force/1 -> Delay/1
  Add2/1 -> Gain2/1
  Band-Limited White Noise/1 -> Gain3/1
  Acceleration/1 -> Add1/2
  Gain5/1 -> Add2/1
  Position/1 -> Add2/2

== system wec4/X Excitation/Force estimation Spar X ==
  Acceleration : Inport
  Velocity : Inport  Port=2
  Position : Inport  Port=3
  PTO Force : Inport  Port=4
  Add : Sum  Inputs=+++
  Add1 : Sum  Inputs=++|
  Add2 : Sum  Inputs=++|
  Add3 : Sum  Inputs=++|
  Add4 : Sum  Inputs=|+-
  Band-Limited White Noise : simulink/Sources/Band-Limited White Noise  Cov=[0.1]  Ts=simu.dt  seed=[23341]
  Band-Limited White Noise1 : simulink/Sources/Band-Limited White Noise  Cov=[0.1]  Ts=simu.dt  seed=[23341]
  Band-Limited White Noise2 : simulink/Sources/Band-Limited White Noise  Cov=[0.1]  Ts=simu.dt  seed=[23341]
  Delay : Delay  DelayLength=1  SampleTime=simu.dt
  Gain : Gain  Gain=rAccelerationGainSparX
  Gain1 : Gain  Gain=rDampingGainSparX
  Gain2 : Gain  Gain=rBuoyancyGainSparX
  Gain3 : Gain  Gain=iSensorNoise
  Gain4 : Gain  Gain=iSensorNoise
  Gain5 : Gain  Gain=iSensorNoise
  To Workspace1 : ToWorkspace  VariableName=arInertialForceSparX  SampleTime=rOutputSampleTime
  To Workspace2 : ToWorkspace  VariableName=accComponentSpH  SampleTime=rOutputSampleTime
  To Workspace3 : ToWorkspace  VariableName=velComponentSpH  SampleTime=rOutputSampleTime
  To Workspace4 : ToWorkspace  VariableName=posComponentSpH  SampleTime=rOutputSampleTime
  Transfer Fcn : TransferFcn  Numerator=arExcForceSparXNum  Denominator=arExcForceSparXDen
  excForce : Outport
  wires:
  Transfer Fcn/1 -> Add4/1, To Workspace1/1
  Add4/1 -> excForce/1
  Add/1 -> Transfer Fcn/1
  Delay/1 -> Add4/2
  Band-Limited White Noise2/1 -> Gain5/1
  Band-Limited White Noise1/1 -> Gain4/1
  Add1/1 -> Gain/1
  Velocity/1 -> Add3/2
  Gain3/1 -> Add1/1
  Add3/1 -> Gain1/1
  Gain4/1 -> Add3/1
  Gain/1 -> Add/1, To Workspace2/1
  Gain1/1 -> To Workspace3/1, Add/2
  Gain2/1 -> To Workspace4/1, Add/3
  PTO Force/1 -> Delay/1
  Add2/1 -> Gain2/1
  Band-Limited White Noise/1 -> Gain3/1
  Acceleration/1 -> Add1/2
  Gain5/1 -> Add2/1
  Position/1 -> Add2/2

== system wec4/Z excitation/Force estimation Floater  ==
  Acceleration : Inport
  Velocity : Inport  Port=2
  Position : Inport  Port=3
  PTO Force : Inport  Port=4
  Add : Sum  Inputs=+++
  Add1 : Sum  Inputs=++|
  Add2 : Sum  Inputs=++|
  Add3 : Sum  Inputs=++|
  Add4 : Sum  Inputs=|+-
  Band-Limited White Noise : simulink/Sources/Band-Limited White Noise  Cov=[0.1]  Ts=simu.dt  seed=[23341]
  Band-Limited White Noise1 : simulink/Sources/Band-Limited White Noise  Cov=[0.1]  Ts=simu.dt  seed=[23341]
  Band-Limited White Noise2 : simulink/Sources/Band-Limited White Noise  Cov=[0.1]  Ts=simu.dt  seed=[23341]
  Delay : Delay  DelayLength=1  SampleTime=simu.dt
  Gain : Gain  Gain=rAccelerationGainFloater
  Gain1 : Gain  Gain=rDampingGainFloater
  Gain2 : Gain  Gain=rBuoyancyGainFloater
  Gain3 : Gain  Gain=iSensorNoise
  Gain4 : Gain  Gain=iSensorNoise
  Gain5 : Gain  Gain=iSensorNoise
  To Workspace1 : ToWorkspace  VariableName=arInertialForceFloater  SampleTime=rOutputSampleTime
  To Workspace2 : ToWorkspace  VariableName=accComponentFl  SampleTime=rOutputSampleTime
  To Workspace3 : ToWorkspace  VariableName=velComponentFl  SampleTime=rOutputSampleTime
  To Workspace4 : ToWorkspace  VariableName=posComponentFl  SampleTime=rOutputSampleTime
  To Workspace5 : ToWorkspace  VariableName=arPtoForce  SampleTime=rOutputSampleTime
  Transfer Fcn : TransferFcn  Numerator=arExcForceFloaterNum  Denominator=arExcForceFloaterDen
  Transfer Fcn1 : TransferFcn  Numerator=arExcForceFloaterNum  Denominator=arExcForceFloaterDen
  Transfer Fcn2 : TransferFcn  Numerator=arExcForceFloaterNum  Denominator=arExcForceFloaterDen
  excForce : Outport
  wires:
  Acceleration/1 -> Add1/2
  Band-Limited White Noise/1 -> Gain3/1
  Add2/1 -> Gain2/1
  PTO Force/1 -> Delay/1
  Gain4/1 -> Add3/1
  Add3/1 -> Gain1/1
  Gain3/1 -> Add1/1
  Velocity/1 -> Add3/2
  Add1/1 -> Gain/1
  Band-Limited White Noise1/1 -> Gain4/1
  Band-Limited White Noise2/1 -> Gain5/1
  Delay/1 -> To Workspace5/1, Add4/2
  Add4/1 -> excForce/1
  Add/1 -> To Workspace1/1, Add4/1
  Transfer Fcn/1 -> Add/2, To Workspace3/1
  Transfer Fcn1/1 -> To Workspace4/1, Add/3
  Gain5/1 -> Add2/1
  Position/1 -> Add2/2
  Gain/1 -> Transfer Fcn2/1
  Gain1/1 -> Transfer Fcn/1
  Gain2/1 -> Transfer Fcn1/1
  Transfer Fcn2/1 -> To Workspace2/1, Add/1

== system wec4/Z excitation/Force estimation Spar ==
  Acceleration : Inport
  Velocity : Inport  Port=2
  Position : Inport  Port=3
  PTO Force : Inport  Port=4
  Add : Sum  Inputs=+++
  Add1 : Sum  Inputs=++|
  Add2 : Sum  Inputs=++|
  Add3 : Sum  Inputs=++|
  Add4 : Sum  Inputs=|+-
  Band-Limited White Noise : simulink/Sources/Band-Limited White Noise  Cov=[0.1]  Ts=simu.dt  seed=[23341]
  Band-Limited White Noise1 : simulink/Sources/Band-Limited White Noise  Cov=[0.1]  Ts=simu.dt  seed=[23341]
  Band-Limited White Noise2 : simulink/Sources/Band-Limited White Noise  Cov=[0.1]  Ts=simu.dt  seed=[23341]
  Gain : Gain  Gain=rAccelerationGainSpar
  Gain1 : Gain  Gain=rDampingGainSpar
  Gain2 : Gain  Gain=rBuoyancyGainSpar
  Gain3 : Gain  Gain=iSensorNoise
  Gain4 : Gain  Gain=iSensorNoise
  Gain5 : Gain  Gain=iSensorNoise
  To Workspace1 : ToWorkspace  VariableName=arInertialForceSpar  SampleTime=rOutputSampleTime
  To Workspace2 : ToWorkspace  VariableName=accComponentSp  SampleTime=rOutputSampleTime
  To Workspace3 : ToWorkspace  VariableName=velComponentSp  SampleTime=rOutputSampleTime
  To Workspace4 : ToWorkspace  VariableName=posComponentSp  SampleTime=rOutputSampleTime
  Transfer Fcn : TransferFcn  Numerator=arExcForceSparNum  Denominator=arExcForceSparDen
  excForce : Outport
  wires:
  Acceleration/1 -> Add1/2
  Band-Limited White Noise/1 -> Gain3/1
  Gain5/1 -> Gain2/1, Add2/1
  Gain2/1 -> To Workspace4/1, Add/3
  Gain1/1 -> To Workspace3/1, Add/2
  Gain/1 -> Add/1, To Workspace2/1
  Gain4/1 -> Add3/1
  Add3/1 -> Gain1/1
  Gain3/1 -> Add1/1
  Velocity/1 -> Add3/2
  Add1/1 -> Gain/1
  Band-Limited White Noise1/1 -> Gain4/1
  Band-Limited White Noise2/1 -> Gain5/1
  PTO Force/1 -> Add4/2
  Add/1 -> Transfer Fcn/1
  Add4/1 -> excForce/1
  Transfer Fcn/1 -> To Workspace1/1, Add4/1
  Position/1 -> Add2/2
